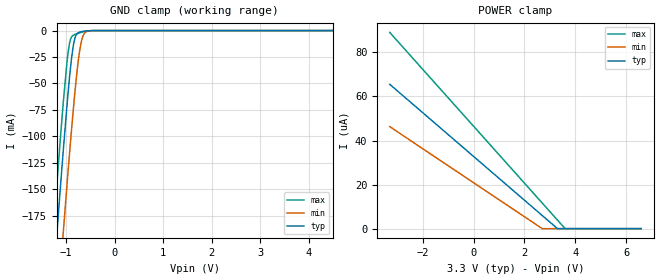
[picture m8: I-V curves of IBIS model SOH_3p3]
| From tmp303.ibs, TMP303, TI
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|   Model
[Model]   SOH_3p3
Model_type   Input
Vinl = 0.99
Vinh = 2.31
|   typ   min   max
C_comp   1pF   1pF   1pF
[Voltage Range]   3.3   2.7   3.6
[Temperature Range]   25   125   -40
[Power Clamp Reference]   3.3   2.7   3.6
[GND Clamp Reference]   -0   -0   -0
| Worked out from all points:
|   GND clamp passes 1 mA (typ) near -0.68 V on its own axis
[GND Clamp]
|   Voltage   I(typ)   I(min)   I(max)
-3.3V     -1.561A    -1.634A    -1.518A
-1.31V    -264.7mA   -343.3mA   -217.6mA
-1.261V   -233.8mA   -312.5mA   -186.7mA
-1.191V   -191.2mA   -269.7mA   -144.1mA
-1.063V   -114.4mA   -191.7mA   -68.86mA
-963.6mV  -59.86mA   -134mA     -21.39mA
-914.1mV  -36.09mA   -106.3mA   -8.589mA
-854.7mV  -14.34mA   -74.86mA   -4.4mA
-735.9mV  -1.704mA   -23.11mA   -2.305mA
-656.7mV  -754.6uA   -5.394mA   -1.282mA
-508.2mV  -81.96uA   -192.3uA   -140.6uA
6.59V     0A         0A         0A
[POWER Clamp]
|   Voltage   I(typ)   I(min)   I(max)
-3.3V     65.53uA    46.32uA    89.08uA
2.689V    6.053uA    70.88nA    11.75uA
3.293V    55.42nA    0A         3.949uA
3.59V     0A         0A         113.9nA
6.59V     0A         0A         0A
